ORGANIZATION_BLOCK MAIN:OB1
TITLE=Ciclo elettropneumatico A+/A-/A+/A-/B+/B-/B+/B-
//Simulatore: 05
//Versione: 1.0
//Data: 28/02/2002
//------------ DESCRIZIONE DEL CONTROLLO ---------------------
// L'esempio utilizza due cilindri (A e B) a doppio effetto e due
// elettrovalvole 5/2 bistabili (1V1 e 2V1).
// Una valvola 3/2 monostabile 0V permette la distribuzione dell'aria al
// circuito.
// Sulla mandata di ciascun cilindro sono preseti degli strozzatori
// unidirezionali che permettono di regolare separatamente la velocità
// delle singole corse dei pistoni.
// Il ciclo continuo inizia con la pressione del pulsante SB1 e potrà
// essere interrotto mediante il pulsante di Stop SB3.
// Il pulsante SB2 permette di resettare i contatori C1 e C2 dei cicli.
// Agli ingressi del PLC vengono collegati:
// - il selettore SA per il comando dell'aria compressa;
// - il pulsante di arresto ciclo SB3;
// - il pulsante di avvio ciclo automatico SB1;
// - i fine corsa magnetici a0, a1, b0, b1 per il controllo
//   della posizione dei pistoni dei cilindri A e B;
// Le segnalazioni sono affidate a due lampade HL1 e HL2 che indicano
// rispettivamente la presenza dell'aria e il ciclo in funzione.

BEGIN
NETWORK 1 //Controllo Distribuzione aria
//
LD I0.0 //S_SB6
= Q0.0 //E_0Y1

NETWORK 2 //Controllo Satrt/Stop Ciclo
//
LD I0.2 //P_SB1
O M0.0 //Ciclo ON
A I0.1 //P_SB3
= M0.0 //Ciclo ON

NETWORK 3 //Contatore cicli A+
//
LD I0.4 //a0
LD C2 //
O I0.3 //P_SB2
CTU C1 +2 //

NETWORK 4 //Contatore Cicli B+
//
LD I0.6 //b0
LD C2 //
O I0.3 //P_SB2
CTU C2 +2 //

NETWORK 5 //Corsa  A+
//
LD M0.0 //Ciclo ON
AN C1 //
A I0.4 //a0
= Q0.1 //E_1Y1

NETWORK 6 //Corsa A-
//
LDN C1 //
A I0.5 //a1
= Q0.2 //E_1Y2

NETWORK 7 //Corsa B+
//
LD I0.6 //b0
AN C2 //
A C1 //
= Q0.3 //E_2Y1

NETWORK 8 //Corsa B-
//
LDN C2 //
A I0.7 //b1
= Q0.4 //E_2Y2

NETWORK 9 //Segnalazione Aria
//
LD Q0.0 //E_0Y1
= Q0.5 //HL1

NETWORK 10 //Segnalazione Ciclo
//
LD M0.0 //CIclo ON
= Q0.6 //HL2

END_ORGANIZATION_BLOCK

